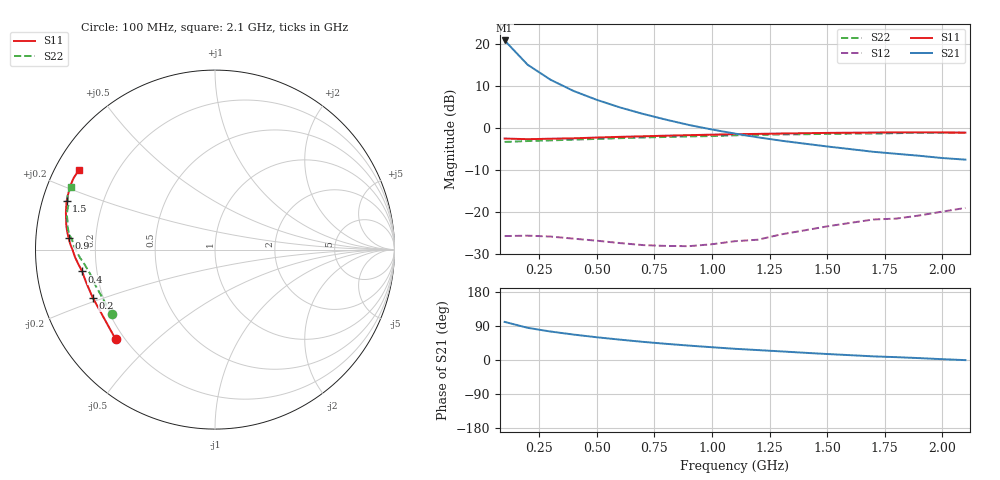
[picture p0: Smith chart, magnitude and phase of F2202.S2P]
! Date: Tue Aug 08 14:31:24 1995
# MHZ  S  MA  R  50.0000
!  POLYFET RF DEVICES
!  F2202
!  S PARAMETERS
!  VDS=28V, IDQ=400mA
!FREQ  S11MAG S11ANG S21MAG S21ANG S12MAG S12ANG S22MAG S22ANG
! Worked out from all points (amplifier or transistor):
!   21 points, 100 MHz to 2.1 GHz, reference 50 ohm
!   highest |S21| = 20.8 dB at 100 MHz (marker M1)
!   |S21| within 3 dB of that: start of sweep to 151.8 MHz
!   unconditionally stable (mu >= 1): 717.2 MHz to 1.383 GHz
!   at 400 MHz: K = 0.52, MSG = 17.6 dB, |S12| = -26.4 dB
!   at 1.1 GHz: K = 1.19, MAG = 10.2 dB, |S12| = -27.0 dB
!   at 2.1 GHz: K = 0.56, MSG = 5.8 dB, |S12| = -19.1 dB
!   S11 on the Smith chart (normalised r, x): 100 MHz: 0.17, -0.37; 200 MHz: 0.16, -0.19; 400 MHz: 0.14, -0.08; 900 MHz: 0.10, +0.04; 1.5 GHz: 0.07, +0.16; 2.1 GHz: 0.07, +0.27
100  0.7453 -138.0  11.02 100.6  0.05116 16.2  0.6789 -147.8
200  0.732 -158.5  5.655 84.9  0.05174 5.7  0.6956 -163.4
300  0.7417 -166.2  3.738 75.1  0.05046 2.4  0.7082 -168.8
400  0.7498 -170.7  2.748 67.1  0.04764 1.1  0.7228 -172.0
500  0.7658 -173.9  2.157 60.0  0.04502 1.5  0.7374 -174.5
600  0.7806 -176.8  1.754 53.8  0.04221 4.0  0.7527 -176.4
700  0.7923 -179.7  1.468 47.9  0.03993 7.6  0.7667 -178.5
800  0.8061 178.0  1.252 42.7  0.03902 13.5  0.7777 179.7
900  0.8177 175.6  1.082 38.0  0.03876 18.3  0.7902 178.0
1000  0.8289 173.2  0.9547 33.7  0.04088 27.6  0.7973 176.1
1100  0.8397 170.7  0.8536 29.5  0.04443 33.3  0.8134 174.4
1200  0.847 168.3  0.7694 26.1  0.04633 37.1  0.8242 172.6
1300  0.8555 166.2  0.7025 22.7  0.05358 41.1  0.8337 170.5
1400  0.8626 163.9  0.6483 19.2  0.05971 42.1  0.8377 168.8
1500  0.8699 161.7  0.5991 15.8  0.06678 41.8  0.848 166.8
1600  0.8744 159.4  0.5577 12.8  0.07346 42.5  0.8516 164.8
1700  0.8782 157.3  0.5179 9.6  0.08064 40.1  0.8534 163.2
1800  0.8814 155.3  0.4902 7.5  0.08266 39.6  0.863 162.0
1900  0.8829 153.1  0.4642 5.0  0.09006 39.2  0.8742 160.0
2000  0.8803 151.2  0.4361 2.1  0.1001 37.6  0.8752 158.0
2100  0.8768 149.5  0.4175 -0.3  0.1108 32.3  0.8734 156.4
